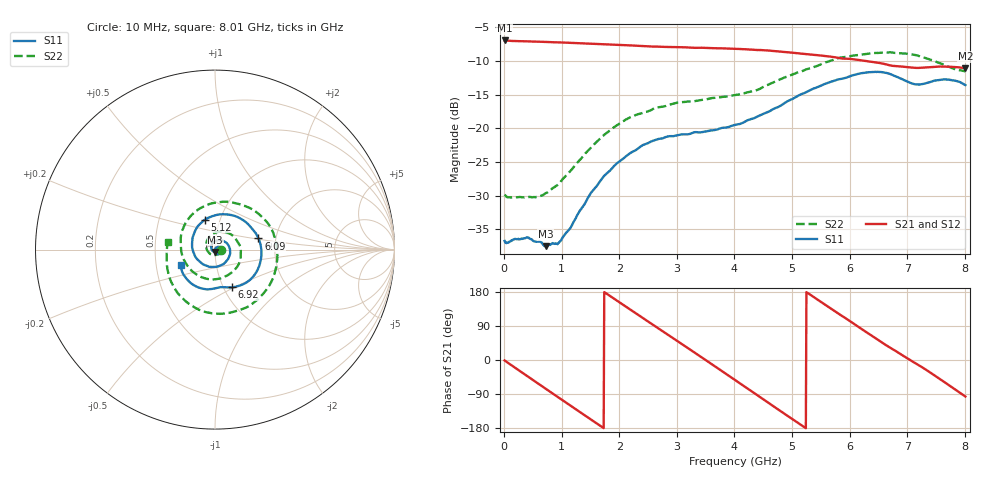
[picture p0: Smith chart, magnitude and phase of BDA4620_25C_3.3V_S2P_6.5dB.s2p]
!Agilent Technologies,E5071B,MY42404982,A.09.10
!Date: Wed May 06 08:49:42 2026
!Data & Calibration Information:
!Freq	S11:SOLT2(ON)	S21:SOLT2(ON)	S12:SOLT2(ON)	S22:SOLT2(ON)
# Hz S RI R 50
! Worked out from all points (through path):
!   801 points, 10 MHz to 8.01 GHz, reference 50 ohm
!   highest |S21| = -6.94 dB at 10 MHz (marker M1); lowest = -11.1 dB at 8.01 GHz (marker M2)
!   group delay of S21, straight-line fit = 283 ps
!   lowest |S11| = -37.5 dB at 720 MHz (marker M3), VSWR 1.03, Z = 50.1 - j1.32 ohm
!   |S11| at or under -10 dB: start of sweep to end of sweep
!   |S22| runs from -30.3 to -8.7 dB; largest |S21 - S12| = 0.0019
!   S11 on the Smith chart (normalised r, x): 10 MHz: 1.03, -0.00; 5.12 GHz: 0.85, +0.29; 6.09 GHz: 1.62, +0.21; 6.92 GHz: 1.10, -0.49; 8.01 GHz: 0.67, -0.12
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1e7  0.0145 -0.00085  0.4499 -0.00961  0.4503 -0.00983  0.032 -0.00246
3.4e8  0.0133 -0.00742  0.3599 -0.26  0.36 -0.2605  0.0203 -0.023
7.2e8  0.0016 -0.0132  0.1101 -0.4248  0.1098 -0.4253  -0.0127 -0.0303
9.7e8  -0.011 -0.00925  -0.086 -0.4263  -0.0864 -0.4267  -0.0365 -0.0147
1.35e9  -0.0214 0.014  -0.3318 -0.2715  -0.3319 -0.2716  -0.0486 0.0357
1.64e9  -0.0117 0.0371  -0.4175 -0.0697  -0.4179 -0.0697  -0.0247 0.0778
1.94e9  0.0143 0.052  -0.3893 0.1515  -0.3898 0.152  0.0281 0.1002
2.32e9  0.0561 0.0425  -0.2039 0.3567  -0.2044 0.3569  0.1041 0.0729
2.68e9  0.0832 0.00381  0.0465 0.4019  0.0471 0.4022  0.1432 0.000889
2.99e9  0.0781 -0.0413  0.2476 0.3163  0.2481 0.3162  0.1341 -0.0766
3.38e9  0.0383 -0.0848  0.3882 0.0838  0.3887 0.0833  0.0542 -0.1516
3.69e9  -0.0127 -0.0968  0.3711 -0.1324  0.3706 -0.1332  -0.044 -0.1629
4.01e9  -0.0701 -0.0793  0.236 -0.3104  0.2358 -0.3109  -0.141 -0.1068
4.52e9  -0.1277 0.0173  -0.1024 -0.3662  -0.1031 -0.3666  -0.1893 0.0787
5.12e9  -0.0568 0.1665  -0.3522 -0.0771  -0.3526 -0.0764  0.000798 0.2617
5.35e9  0.0156 0.1947  -0.3457 0.0679  -0.3457 0.0685  0.1122 0.2591
5.73e9  0.1508 0.1678  -0.2172 0.2596  -0.2172 0.2601  0.2792 0.1655
6.09e9  0.2423 0.0621  -0.0215 0.3244  -0.0208 0.3248  0.3477 -0.0212
6.68e9  0.1817 -0.1792  0.243 0.1676  0.2442 0.1674  0.2 -0.3074
6.92e9  0.0959 -0.2099  0.2809 0.0606  0.2819 0.06  0.0695 -0.3542
7.48e9  -0.0478 -0.2212  0.2162 -0.1873  0.2164 -0.1883  -0.2165 -0.2291
8.01e9  -0.1909 -0.0862  -0.0311 -0.2777  -0.0318 -0.2786  -0.2618 0.0396
